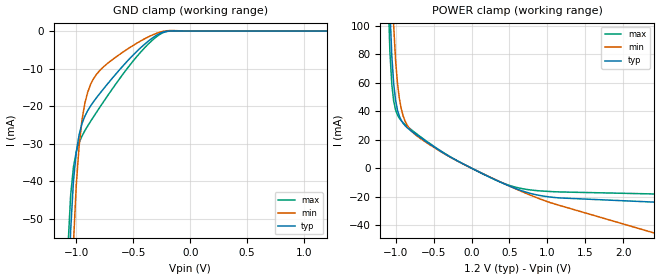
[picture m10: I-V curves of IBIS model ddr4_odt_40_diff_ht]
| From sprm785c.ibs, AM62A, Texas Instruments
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|   Model ddr4_odt_40_diff_ht
[Model] ddr4_odt_40_diff_ht
Model_type Input
Polarity   Non-Inverting
Enable   Active-High
Vinl =  0.700V
Vinh =  0.900V
C_comp   2.181pF   2.106pF   2.362pF
[Model Spec]
Vinh   0.900V   0.820V   0.980V
Vinl   0.700V   0.620V   0.780V
[Temperature Range]   25.000   0.125k   -40.000
[Voltage Range]   1.200V   1.140V   1.260V
[C Comp Corner]
C_comp   2.181pF   2.106pF   2.362pF
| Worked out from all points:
|   GND clamp passes 1 mA (typ) near -0.29 V on its own axis
|   POWER clamp passes 1 mA (typ) near -0.04 V on its own axis
[GND_clamp]
|Voltage   I(typ)   I(min)   I(max)
-1.2V     -384.2mA   -427.1mA   -361.3mA
-1.075V   -75.51mA   -111.4mA   -58.73mA
-1.05V    -53.29mA   -79.39mA   -43.81mA
-1.025V   -39.9mA    -56.5mA    -36.16mA
-1V       -32.1mA    -40.83mA   -32.11mA
-975mV    -27.5mA    -30.44mA   -29.67mA
-925mV    -22.67mA   -19.22mA   -26.53mA
-825mV    -17.84mA   -11.62mA   -21.72mA
-650mV    -11.34mA   -6.873mA   -13.96mA
-400mV    -3.498mA   -2.058mA   -4.46mA
-225mV    -185.2uA   -12.61uA   -274.2uA
1.2V      0A         0A         0A
[POWER_clamp]
|Voltage   I(typ)   I(min)   I(max)
-1.2V     599.9mA    739.5mA    627.1mA
-1.1V     163.3mA    255.3mA    125.5mA
-1.075V   111.9mA    186.1mA    81.9mA
-1.05V    79.07mA    135.3mA    58.84mA
-1.025V   59.3mA     99.77mA    47.11mA
-1V       47.67mA    75.61mA    40.91mA
-975mV    40.74mA    59.49mA    37.31mA
-925mV    33.51mA    41.57mA    33.27mA
-825mV    27.41mA    28.28mA    28.4mA
-325mV    9.238mA    9.08mA     9.428mA
675mV     -16.11mA   -16.72mA   -14.46mA
2.4V      -23.84mA   -45.45mA   -18.12mA
